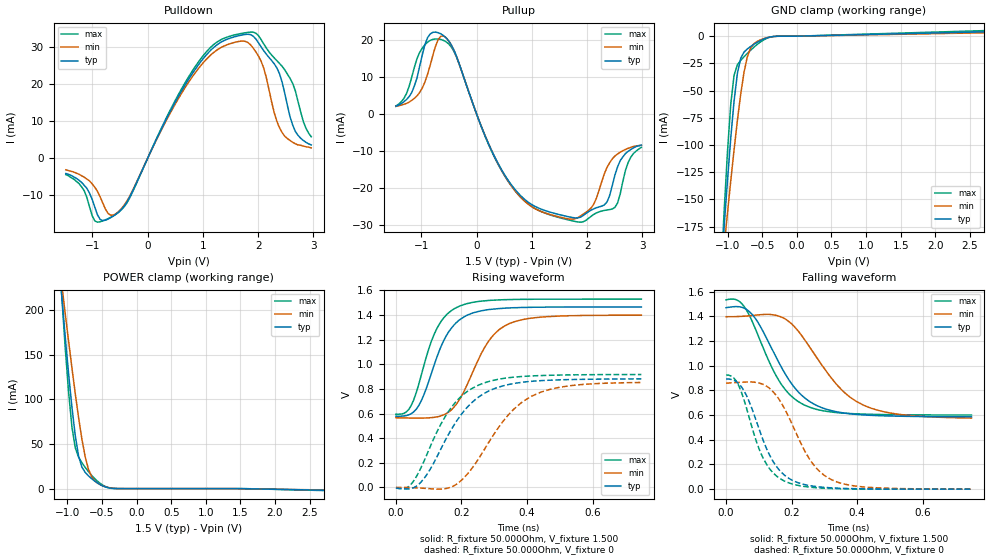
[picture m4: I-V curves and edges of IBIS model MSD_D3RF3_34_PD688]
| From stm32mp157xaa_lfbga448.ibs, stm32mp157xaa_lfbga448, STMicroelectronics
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[Model] MSD_D3RF3_34_PD688
Model_type   I/O
C_comp 2.444pF   2.361pF   2.568pF
Vinh = 925.000mV
Vinl = 575.000mV
Vmeas = 750.000mV
Vref = 750.000mV
[Model Spec]
Vinh   925.000mV   888.000mV   963.000mV
Vinl   575.000mV   538.000mV   613.000mV
Vmeas   750.000mV   713.000mV   788.000mV
Vref   750.000mV   713.000mV   788.000mV
[Temperature Range]   25.000   125.000   -40.000
[Voltage Range]   1.500V   1.425V   1.575V
[GND Clamp Reference]   0.00V   0.00V   0.00V
[Pulldown Reference]   0.00V   0.00V   0.00V
[POWER Clamp Reference]   1.500V   1.425V   1.575V
[Pullup Reference]   1.500V   1.425V   1.575V
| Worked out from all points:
|   slope of the pulldown table from 0 to 0.225 V, typ, clamps not added: 31.5 ohm
|   slope of the pullup table from 0 to 0.225 V, typ, clamps not added: 26.9 ohm
|   GND clamp passes 1 mA (typ) near -0.40 V on its own axis
|   POWER clamp passes 1 mA (typ) near -0.41 V on its own axis
|   rising waveform, R_fixture 50.000Ohm, V_fixture 1.500: 20-80 % time 82.1ps typ, 97.8ps min, 73.1ps max; typ from 0.578 V to 1.46 V
|   rising waveform, R_fixture 50.000Ohm, V_fixture 0: 20-80 % time 128ps typ, 144ps min, 117ps max; typ from -0.005 V to 0.881 V
|   falling waveform, R_fixture 50.000Ohm, V_fixture 1.500: 20-80 % time 120ps typ, 147ps min, 105ps max; typ from 1.47 V to 0.586 V
|   falling waveform, R_fixture 50.000Ohm, V_fixture 0: 20-80 % time 85.7ps typ, 104ps min, 75ps max; typ from 0.893 V to 0 V
[GND Clamp]
-1.48V    -595.2mA   -480.8mA   -764.9mA
-1.098V   -219.1mA   -224mA     -221.3mA
-1.05V    -174.8mA   -193mA     -160.6mA
-1.002V   -132.6mA   -162.5mA   -106.1mA
-954.6mV  -93.48mA   -132.9mA   -62.36mA
-906.8mV  -59.6mA    -104.4mA   -35.9mA
-859.1mV  -34.32mA   -77.6mA    -26.31mA
-811.4mV  -20.37mA   -53.46mA   -22.22mA
-715.9mV  -11.76mA   -19.03mA   -15.86mA
-572.7mV  -5.614mA   -4.804mA   -7.58mA
-286.4mV  -74.25uA   -124.6uA   -59.77uA
2.959V    4.342mA    3.42mA     5.581mA
[Power Clamp]
-1.459V   578.9mA    480.2mA    724.6mA
-1.077V   211.8mA    226.1mA    211.3mA
-1.03V    168.9mA    195.3mA    156.5mA
-981.8mV  128.3mA    164.9mA    107.6mA
-934.1mV  91.11mA    135.2mA    69.06mA
-886.4mV  59.57mA    106.6mA    45.9mA
-838.6mV  36.67mA    79.82mA    35.26mA
-743.2mV  18.24mA    35.86mA    23.8mA
-647.7mV  11.02mA    13.07mA    14.69mA
-552.3mV  5.649mA    5.582mA    7.444mA
-313.6mV  104.8uA    243.3uA    121.9uA
2.98V     -2.208mA   -1.853mA   -2.682mA
[Pulldown]
-1.48V    -4.1mA     -3.1mA     -4.4mA
-1.145V   -7.3mA     -5.1mA     -8.8mA
-954.6mV  -13.2mA    -7.8mA     -16.87mA
-811.4mV  -16.78mA   -12.04mA   -16.85mA
-572.7mV  -15.06mA   -14.9mA    -15.04mA
-334.1mV  -10.72mA   -10.48mA   -10.95mA
906.8mV   24.92mA    23.93mA    25.67mA
1.766V    33.34mA    31.48mA    33.8mA
2.052V    30.01mA    26.15mA    31.98mA
2.434V    20.41mA    6.9mA      24.74mA
2.673V    7.2mA      3.9mA      18.1mA
2.959V    3.6mA      2.8mA      5.8mA
[Pullup]
-1.459V   2.1mA      2.057mA    2.171mA
-1.03V    12.9mA     5.828mA    16.66mA
-886.4mV  20.67mA    10.76mA    19.45mA
-647.7mV  21.69mA    21.03mA    20.17mA
-409.1mV  17.29mA    17.18mA    16.92mA
211.4mV   -7.901mA   -7.87mA    -8.056mA
688.6mV   -20.3mA    -20.62mA   -20.64mA
1.834V    -28.1mA    -28.01mA   -29.21mA
2.359V    -23.78mA   -14.44mA   -25.96mA
2.502V    -16.5mA    -11.36mA   -25.27mA
2.741V    -10.1mA    -9.286mA   -13.11mA
2.98V     -8.4mA     -8.443mA   -9.029mA
[Ramp]
R_load=50.000Ohm
dV/dt_r   527.970mV/106.000ps  504.839mV/122.000ps  552.990mV/95.500ps
dV/dt_f   527.970mV/103.500ps  504.809mV/127.500ps  552.990mV/91.000ps
[Rising waveform]
R_fixture=50.000Ohm
V_fixture=1.500
V_fixture_min=1.425
V_fixture_max=1.575
0s        577.9mV    565.7mV    594.2mV
39ps      588.6mV    563.4mV    632.7mV
69ps      661.4mV    562.7mV    830.6mV
123ps     1.042V     571.8mV    1.279V
154ps     1.232V     599.9mV    1.4V
192ps     1.355V     704.9mV    1.468V
276ps     1.44V      1.159V     1.515V
345ps     1.456V     1.328V     1.524V
460ps     1.463V     1.385V     1.527V
749ps     1.464V     1.397V     1.528V
[Rising waveform]
R_fixture=50.000Ohm
V_fixture=0
0s        -4.986mV   829.3uV    -5.146mV
39ps      -11.61mV   -839uV     7.709mV
77ps      45.04mV    -5.082mV   162.8mV
161ps     433mV      -2.958mV   618.5mV
207ps     617.7mV    76.97mV    756.7mV
253ps     734.9mV    236.4mV    831.2mV
345ps     835.5mV    595mV      890.4mV
414ps     860.9mV    740.2mV    904.6mV
529ps     875mV      824.3mV    913mV
749ps     880.8mV    851.5mV    916.1mV
[Falling waveform]
R_fixture=50.000Ohm
V_fixture=1.500
V_fixture_min=1.425
V_fixture_max=1.575
0s        1.47V      1.397V     1.534V
46ps      1.475V     1.4V       1.509V
85ps      1.399V     1.408V     1.327V
161ps     1.027V     1.402V     881.5mV
199ps     858.5mV    1.342V     754.5mV
238ps     743.8mV    1.217V     683.1mV
337ps     627.3mV    849.2mV    620.6mV
421ps     601.1mV    678.5mV    608mV
529ps     591.1mV    605.8mV    602.6mV
749ps     586.2mV    576.2mV    600.9mV
[Falling waveform]
R_fixture=50.000Ohm
V_fixture=0
0s        892.8mV    858.6mV    925.1mV
31ps      871.8mV    863.6mV    876.8mV
54ps      800.7mV    867.3mV    730.8mV
115ps     384.1mV    846.8mV    241.8mV
146ps     213.6mV    782.1mV    125.7mV
177ps     116.4mV    659.3mV    67.41mV
261ps     26.47mV    218.9mV    14.96mV
330ps     9.549mV    67.34mV    4.67mV
444ps     1.977mV    13.36mV    725.8uV
749ps     63.3uV     469.6uV    -7.644uV
